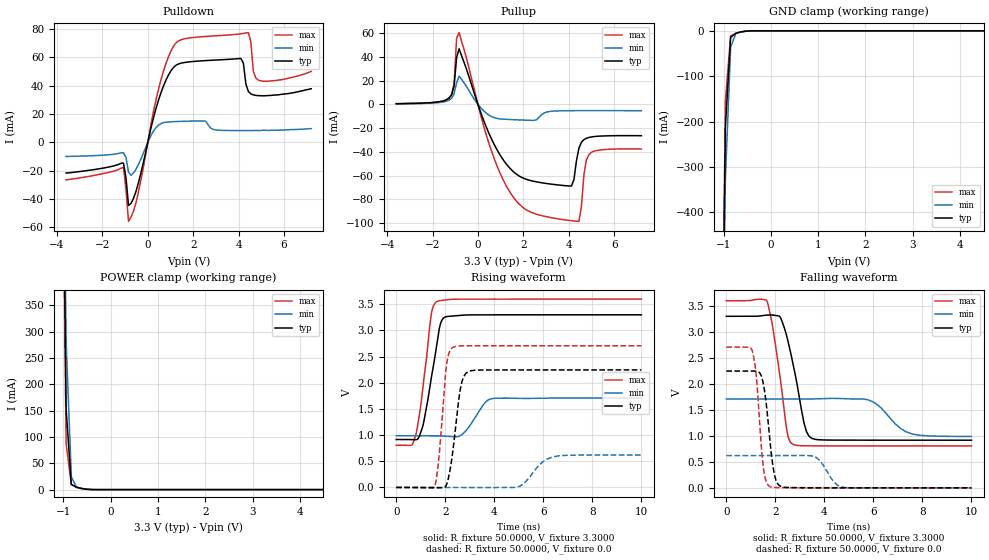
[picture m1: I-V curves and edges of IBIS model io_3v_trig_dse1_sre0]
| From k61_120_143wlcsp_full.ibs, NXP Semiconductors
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[Model]  io_3v_trig_dse1_sre0
|   Model io_3v_trig_dse1_sre0
| Library cells for typ/min/max conditions are connected as defined below:
|  pad - External Pad
|  ipp_do_3v - Core Input
|  ipp_obe_3v - Output Buffer Enable
|  esd_boost - vdd_s_3v
|  esd_trigger - vss_s_3v
|  ipp_ame_3v - vss_s_3v
|  ipp_dse_3v - vdd_s_3v
|  ipp_ina_3v - NC
|  ipp_ina_mux_3v - NC
|  ipp_ind_3v - NC
|  ipp_pue_3v - vss_s_3v
|  ipp_sre_3v - vss_s_3v
|  tie_3v - vdd_s_3v
|  tie_hi - vdd_s_lv
|  vbuf_3v - vdd_s_3v
|  vdd_s_3v - vdd_s_3v
|  vdd_s_lv - vdd_s_lv
|  vss_bulk - vss_s_3v
|  vss_s_3v - vss_s_3v
| All other pins connected to ground
Model_type I/O
Polarity   Non-Inverting
Enable   Active-High
Vinl =   1.1550V
Vinh =   2.3100V
Vmeas =  1.6500V
Cref =   25.0000pF
Rref =   50.0000
Vref =   0.0V
C_comp   1.9033pF   1.7921pF   2.1182pF
[Temperature Range]   25.0000   0.1250k   -40.0000
[Voltage Range]   3.3000V   1.7100V   3.6000V
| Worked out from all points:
|   slope of the pulldown table from 0 to 0.495 V, typ, clamps not added: 16 ohm
|   slope of the pullup table from 0 to 0.495 V, typ, clamps not added: 19.9 ohm
|   GND clamp passes 1 mA (typ) near -0.54 V on its own axis
|   POWER clamp passes 1 mA (typ) near -0.53 V on its own axis
|   rising waveform, R_fixture 50.0000, V_fixture 3.3000: 20-80 % time 500ps typ, 602ps min, 420ps max; typ from 0.916 V to 3.3 V
|   rising waveform, R_fixture 50.0000, V_fixture 0.0: 20-80 % time 352ps typ, 691ps min, 276ps max; typ from 0 V to 2.25 V
|   falling waveform, R_fixture 50.0000, V_fixture 3.3000: 20-80 % time 594ps typ, 898ps min, 484ps max; typ from 3.3 V to 0.917 V
|   falling waveform, R_fixture 50.0000, V_fixture 0.0: 20-80 % time 311ps typ, 515ps min, 259ps max; typ from 2.25 V to 0 V
[Pulldown]
|Voltage   I(typ)   I(min)   I(max)
-3.6V     -21.69mA   -9.96mA    -26.46mA
-1.07V    -14.69mA   -7.404mA   -17.65mA
-850mV    -44.53mA   -20.93mA   -55.69mA
-520mV    -34.62mA   -18.99mA   -42.62mA
580mV     34.99mA    13.27mA    44.1mA
1.46V     55.81mA    14.79mA    72.31mA
4.1V      59.15mA    8.3mA      76.57mA
4.43V     35.88mA    8.3mA      77.43mA
4.54V     34.19mA    8.3mA      70.65mA
4.65V     33.46mA    8.3mA      49.92mA
4.87V     32.94mA    8.3mA      43.91mA
7.2V      37.8mA     9.7mA      50mA
[Pullup]
|Voltage   I(typ)   I(min)   I(max)
-3.6V     600uA      400uA      600uA
-1.27V    5.28mA     3.56mA     5.35mA
-1.05V    15.3mA     8.87mA     17.35mA
-940mV    39.22mA    18.09mA    55.5mA
-830mV    46.74mA    23.72mA    60.38mA
1.15V     -47.61mA   -12.48mA   -64.99mA
3.24V     -67.13mA   -5.816mA   -95.35mA
4.12V     -68.69mA   -5.32mA    -97.87mA
4.45V     -36.82mA   -5.29mA    -98.37mA
4.78V     -28.52mA   -5.28mA    -46.64mA
5V        -27.41mA   -5.28mA    -40.35mA
7.2V      -26.38mA   -5.36mA    -37.57mA
[GND_clamp]
|Voltage   I(typ)   I(min)   I(max)
-3.6V     -47.82A    -47.1A     -48.34A
-1.07V    -1.102A    -1.183A    -1.105A
-960mV    -210.7mA   -326mA     -154mA
-850mV    -14.47mA   -36.11mA   -11.11mA
-740mV    -5.262mA   -6.033mA   -5.843mA
-520mV    -636.9uA   -915.4uA   -467.5uA
-300mV    -2.578uA   -18.09uA   -370.9nA
7.2V      0A         0A         0A
[POWER_clamp]
|Voltage   I(typ)   I(min)   I(max)
-3.6V     36.98A     36.74A     37.19A
-1.05V    1.02A      1.161A     949.9mA
-940mV    152.3mA    280.6mA    87.35mA
-830mV    9.987mA    24.48mA    9.181mA
-720mV    4.227mA    4.408mA    5.116mA
-500mV    628.6uA    743.9uA    622.6uA
-390mV    66.57uA    164uA      29.9uA
7.2V      0A         0A         0A
[Ramp]
| variable   typ   min   max
dV/dt_r  1.3476/0.3518n   0.3718/0.6914n   1.6250/0.2756n
dV/dt_f  1.4298/0.5936n   0.4329/0.8979n   1.6761/0.4835n
R_load = 50.0000
[Rising Waveform]
R_fixture= 50.0000
V_fixture= 3.3000
V_fixture_min= 1.7100
V_fixture_max= 3.6000
|time   V(typ)   V(min)   V(max)
0s        916.5mV    987.1mV    806.1mV
655.6ps   914.3mV    987.1mV    817.1mV
816.4ps   912.4mV    987.2mV    1.035V
1.097ns   1.192V     987.7mV    1.946V
1.408ns   2.029V     987.2mV    3.239V
1.649ns   2.723V     985.9mV    3.551V
1.956ns   3.247V     981.5mV    3.582V
2.712ns   3.293V     1.019V     3.599V
3.864ns   3.3V       1.694V     3.599V
10ns      3.3V       1.71V      3.6V
[Rising Waveform]
R_fixture= 50.0000
V_fixture= 0.0
V_fixture_min= 0.0
V_fixture_max= 0.0
|time   V(typ)   V(min)   V(max)
0s        2.009nV    218.2nV    1.41nV
1.573ns   -4.871mV   12.4uV     29.97mV
1.723ns   -7.154mV   20.78uV    480.4mV
2.064ns   65.73mV    61.66uV    2.383V
2.334ns   784.5mV    46.86uV    2.683V
2.608ns   1.862V     -610.4uV   2.705V
2.94ns    2.214V     -1.558mV   2.708V
4.97ns    2.246V     11.93mV    2.708V
6.38ns    2.246V     583mV      2.708V
10ns      2.246V     619.6mV    2.708V
[Falling Waveform]
R_fixture= 50.0000
V_fixture= 3.3000
V_fixture_min= 1.7100
V_fixture_max= 3.6000
|time   V(typ)   V(min)   V(max)
0s        3.3V       1.71V      3.6V
1.646ns   3.323V     1.71V      3.603V
2.22ns    3.267V     1.71V      2.032V
2.517ns   2.817V     1.71V      986mV
2.682ns   2.471V     1.71V      846.2mV
3.165ns   1.254V     1.71V      809.3mV
3.49ns    952.4mV    1.711V     808mV
5.794ns   917.3mV    1.691V     806.7mV
7.592ns   917.1mV    1.035V     806.6mV
10ns      917mV      988.5mV    806.6mV
[Falling Waveform]
R_fixture= 50.0000
V_fixture= 0.0
V_fixture_min= 0.0
V_fixture_max= 0.0
|time   V(typ)   V(min)   V(max)
0s        2.246V     620mV      2.709V
1.053ns   2.247V     619.9mV    2.643V
1.201ns   2.247V     619.9mV    2.25V
1.492ns   2.043V     619.8mV    466.6mV
1.756ns   1.018V     619.8mV    28.76mV
1.97ns    236.5mV    619.9mV    7.226mV
2.289ns   16.04mV    620.1mV    4.412mV
3.657ns   547.9uV    586.8mV    394.5uV
4.799ns   326.1uV    9.356mV    349.7uV
10ns      246uV      111.4uV    266.9uV
